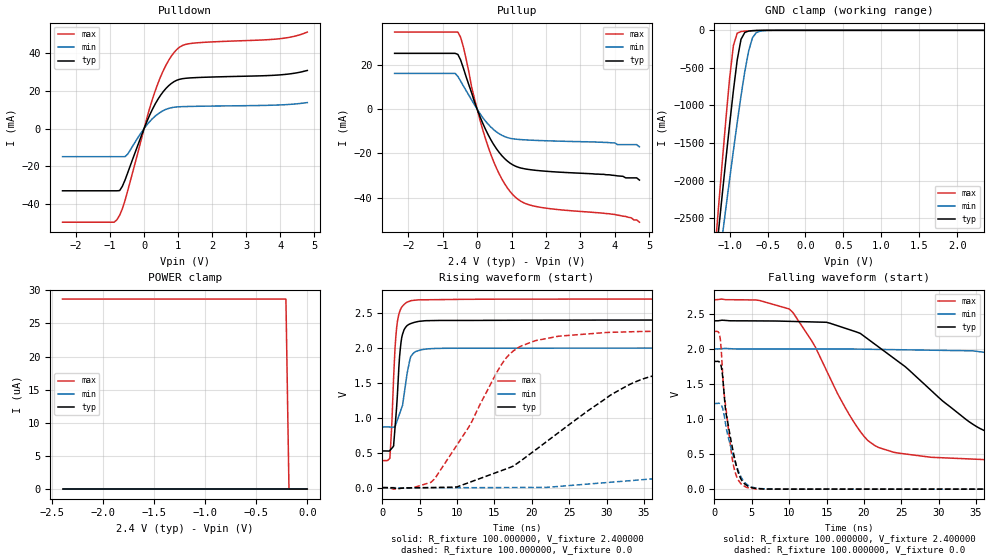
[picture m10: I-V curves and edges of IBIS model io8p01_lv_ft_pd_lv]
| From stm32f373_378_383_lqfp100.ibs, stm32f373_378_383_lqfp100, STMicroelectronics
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|   Model io8p01_lv_ft_pd_lv
[Model]  io8p01_lv_ft_pd_lv
Model_type I/O
Polarity   Non-Inverting
Enable   Active-Low
Vinl =   0.720000V
Vinh =   1.680000V
Vmeas =  1.200000V
Cref =   50.000000pF
Rref =   100.000000M
Vref =   0.0V
C_comp   5.024800pF   4.846300pF   5.260300pF
[Temperature Range]   25.000000   0.125000k   -40.000000
[Pullup Reference]   2.400000V   2.000000V   2.700000V
[Pulldown Reference]   0.0V   0.0V   0.0V
[POWER Clamp Reference]   2.400000V   2.000000V   2.700000V
[GND Clamp Reference]   0.0V   0.0V   0.0V
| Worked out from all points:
|   slope of the pulldown table from 0 to 0.36 V, typ, clamps not added: 25.5 ohm
|   slope of the pullup table from 0 to 0.36 V, typ, clamps not added: 28.4 ohm
|   GND clamp passes 1 mA (typ) near -0.60 V on its own axis
|   rising waveform, R_fixture 100.000000, V_fixture 2.400000: 20-80 % time 715ps typ, 1.15ns min, 634ps max; typ from 0.525 V to 2.4 V
|   rising waveform, R_fixture 100.000000, V_fixture 0.0: 20-80 % time 14.5ns typ, 42.8ns min, 7.19ns max; typ from 0 V to 1.82 V
|   falling waveform, R_fixture 100.000000, V_fixture 2.400000: 20-80 % time 13ns typ, 31.4ns min, 7.08ns max; typ from 2.4 V to 0.525 V
|   falling waveform, R_fixture 100.000000, V_fixture 0.0: 20-80 % time 1.64ns typ, 1.84ns min, 1.35ns max; typ from 1.82 V to 0 V
[Pulldown]
|Voltage   I(typ)   I(min)   I(max)
-2.4V     -33.16mA   -14.98mA   -49.86mA
-880mV    -33.16mA   -14.98mA   -49.86mA
-800mV    -33.16mA   -14.98mA   -48.55mA
-640mV    -30.75mA   -14.98mA   -42.77mA
-480mV    -23.43mA   -13.57mA   -32.92mA
80mV      3.651mA    1.905mA    5.506mA
400mV     15.37mA    7.665mA    23.73mA
720mV     22.75mA    10.69mA    36.23mA
1.04V     26.18mA    11.57mA    43.27mA
1.52V     27.09mA    11.81mA    45.55mA
4V        28.55mA    12.55mA    47.81mA
4.8V      30.9mA     13.81mA    51.31mA
[Pullup]
|Voltage   I(typ)   I(min)   I(max)
-2.4V     25.18mA    16.13mA    34.78mA
-640mV    25.18mA    16.13mA    34.78mA
-560mV    24.71mA    14.76mA    34.78mA
-400mV    18.52mA    10.49mA    28.1mA
-160mV    7.343mA    4.152mA    10.02mA
80mV      -3.229mA   -1.94mA    -4.736mA
400mV     -13.82mA   -8.08mA    -20.45mA
800mV     -22.31mA   -12.38mA   -33.66mA
1.2V      -26.24mA   -13.65mA   -40.82mA
1.76V     -27.69mA   -14.12mA   -44.06mA
4V        -29.9mA    -15.2mA    -47.5mA
4.72V     -32mA      -17mA      -51mA
[GND_clamp]
|Voltage   I(typ)   I(min)   I(max)
-2.4V     -9.914A    -9.862A    -9.419A
-1.2V     -3.21A     -3.567A    -3.02A
-1.15V    -2.709A    -3.165A    -2.399A
-1.1V     -2.213A    -2.766A    -1.788A
-1.05V    -1.726A    -2.371A    -1.195A
-950mV    -800.5mA   -1.599A    -202.1mA
-900mV    -395mA     -1.228A    -38.18mA
-850mV    -120.2mA   -874.5mA   -15.93mA
-750mV    -9.822mA   -279.4mA   -7.289mA
-700mV    -4.75mA    -102mA     -4.527mA
-600mV    -1.046mA   -11.1mA    -938uA
2.35V     59.64uA    46.24uA    66.77uA
[POWER_clamp]
|Voltage   I(typ)   I(min)   I(max)
-2.4V     0A         0A         28.66uA
-210mV    0A         0A         28.66uA
-180mV    0A         0A         0A
0V        0A         0A         0A
[Ramp]
| variable   typ   min   max
dV/dt_r  1.09212/14.44718n   0.73278/42.74614n   1.34886/7.17215n
dV/dt_f  1.12427/12.94219n   0.67775/31.41448n   1.38695/7.06999n
R_load = 100.000000
[Rising Waveform]
R_fixture= 100.000000
V_fixture= 2.400000
V_fixture_min= 2.000000
V_fixture_max= 2.700000
|time   V(typ)   V(min)   V(max)
0s        524.8mV    868.7mV    387.2mV
1.001ns   531.1mV    867.6mV    420mV
1.301ns   567.5mV    866.3mV    1V
1.502ns   596.3mV    865.7mV    1.56V
1.902ns   1.141V     934.9mV    2.28V
2.503ns   2.084V     1.118V     2.567V
3.303ns   2.318V     1.629V     2.654V
4.204ns   2.363V     1.93V      2.681V
6.306ns   2.39V      1.988V     2.689V
49.85ns   2.399V     1.999V     2.699V
[Rising Waveform]
R_fixture= 100.000000
V_fixture= 0.0
V_fixture_min= 0.0
V_fixture_max= 0.0
|time   V(typ)   V(min)   V(max)
0s        4.868nV    72.49nV    3.74nV
6.507ns   464.5uV    -265.9uV   76.76mV
11.51ns   69.9mV     -183.7uV   858.8mV
17.02ns   286.1mV    1.385mV    1.91V
24.02ns   823.7mV    21.3mV     2.172V
34.53ns   1.542V     111.6mV    2.235V
47.05ns   1.754V     293mV      2.246V
83.08ns   1.82V      928.7mV    2.248V
106.1ns   1.82V      1.126V     2.248V
249.2ns   1.82V      1.221V     2.248V
[Falling Waveform]
R_fixture= 100.000000
V_fixture= 2.400000
V_fixture_min= 2.000000
V_fixture_max= 2.700000
|time   V(typ)   V(min)   V(max)
0s        2.399V     1.999V     2.699V
10.01ns   2.391V     1.997V     2.568V
15.02ns   2.378V     1.997V     1.687V
20.52ns   2.14V      1.994V     693.4mV
29.03ns   1.403V     1.98V      454.1mV
37.04ns   797.1mV    1.937V     417.2mV
51.05ns   601.2mV    1.692V     397.2mV
78.08ns   542mV      1.107V     387.8mV
101.6ns   527.4mV    959.8mV    387.2mV
249.2ns   524.8mV    868.7mV    387.2mV
[Falling Waveform]
R_fixture= 100.000000
V_fixture= 0.0
V_fixture_min= 0.0
V_fixture_max= 0.0
|time   V(typ)   V(min)   V(max)
0s        1.82V      1.221V     2.248V
500.5ps   1.821V     1.223V     2.242V
800.8ps   1.79V      1.216V     2.124V
1.101ns   1.603V     1.151V     1.642V
1.301ns   1.348V     1.052V     1.358V
1.502ns   1.114V     921.4mV    1.186V
2.603ns   487.2mV    445.5mV    310.3mV
3.403ns   176mV      208.9mV    97.85mV
4.304ns   55.11mV    70.91mV    24.78mV
49.85ns   4.868nV    72.49nV    3.74nV
